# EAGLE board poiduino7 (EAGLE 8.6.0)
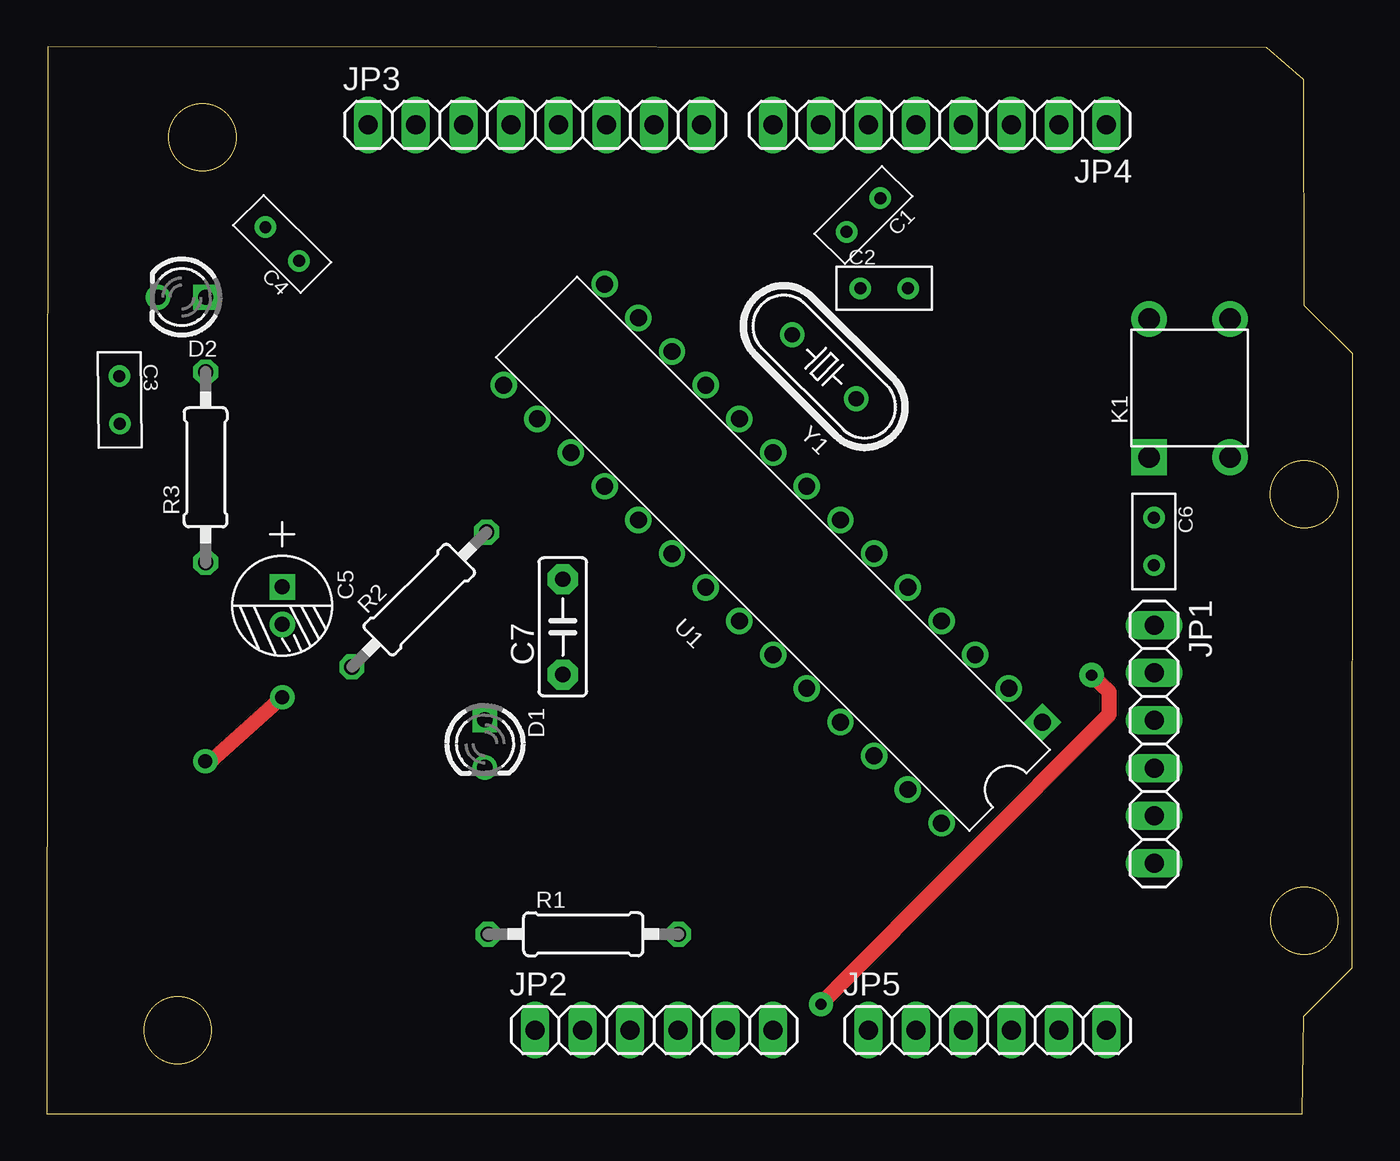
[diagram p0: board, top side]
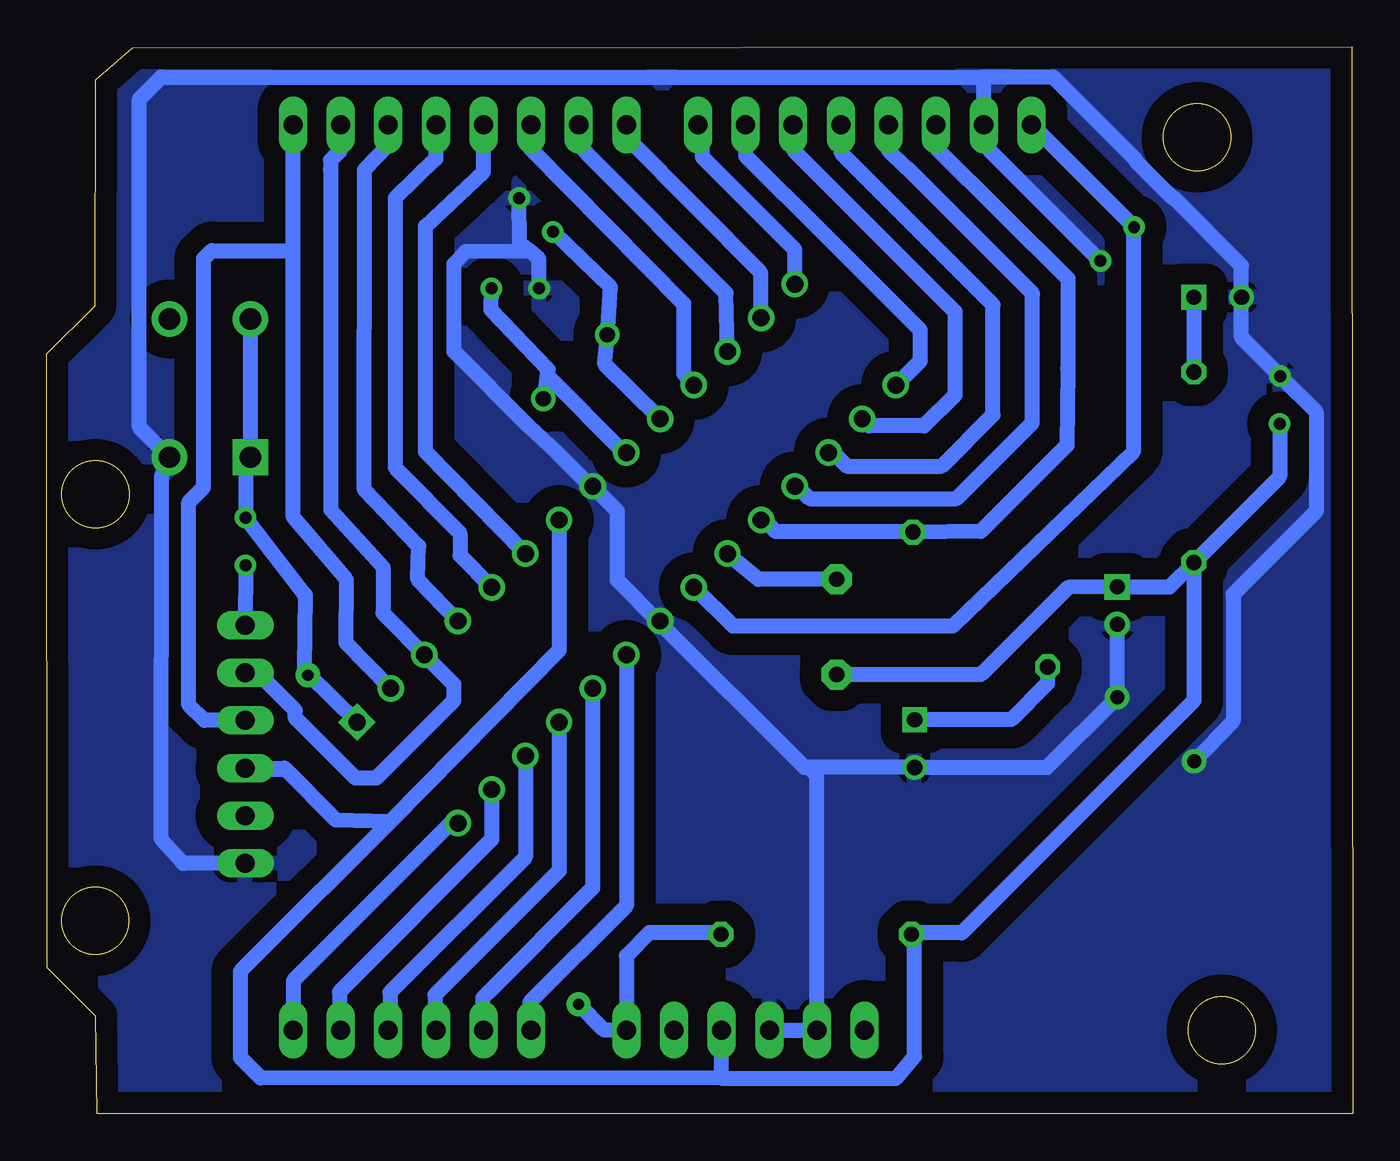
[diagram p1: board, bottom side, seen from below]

Size 69.63 x 56.88 mm. Coordinates in mm from the lower left corner, seen from the top.
Outline: 0,0.01 59.03,0.01 66.95,0 67.02,5.21 69.61,7.8 69.63,40.51 67.06,43.08 67.02,55.14 65.05,56.84 0.05,56.88 0,0.01
Outline: circle at 8.29,52.06 radius 1.8
Outline: circle at 6.98,4.47 radius 1.8
Outline: circle at 67.04,33.04 radius 1.8
Outline: circle at 67.05,10.3 radius 1.8
Copper layers (1*16): Top 0.035mm / dielectric 1.5mm / Bottom 0.035mm
Design rules "default": minimum track width 6mil, minimum drill 0.35mm, track to track 6mil, track to pad 6mil, pad to pad 6mil, via to via 6mil, smd to smd 6mil, copper to edge 40mil, drill to drill 6mil, minimum pad ring 10mil, minimum via ring 8mil, stop-mask expansion 4mil, vias tented up to drill 0mil, thermal gap 10mil

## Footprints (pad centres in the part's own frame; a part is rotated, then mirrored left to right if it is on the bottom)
CERAMIC-2.54 = drill 0.635 pad 1.143: 1 -1.27,0; 2 1.27,0
PC-D5.3MM = drill 0.8 pad 1.35 square: + -1,0 | drill 0.8 pad 1.35: - 1,0
C5B2.5 = drill 0.813 pad 1.6 octagon: 1 -2.54,0; 2 2.54,0
LED2-2.54-D3.0MM = drill 0.813 square: A -1.27,0 | drill 0.813: K 1.27,0
1X06 = drill 1.016 long: 1 -6.35,0; 2 -3.81,0; 3 -1.27,0; 4 1.27,0; 5 3.81,0; 6 6.35,0
1X08 = drill 1.016 long: 1 -8.89,0; 2 -6.35,0; 3 -3.81,0; 4 -1.27,0; 5 1.27,0; 6 3.81,0; 7 6.35,0; 8 8.89,0
SW4-6.0X6.0X5.0MM = drill 1.143 pad 1.905 square: 1 -3.683,2.159 | drill 1.143 pad 1.905: 2 -3.683,-2.159; 3 3.683,-2.159; 4 3.683,2.159
PR-D2.3XL6.5MM = drill 0.813 octagon: 1 -4.953,0; 2 5.207,0
DIP28-2.54-34.7X7.62MM = drill 0.9 pad 1.4 square: 1 -16.51,-3.81 | drill 0.9 pad 1.4: 2 -13.97,-3.81; 3 -11.43,-3.81; 4 -8.89,-3.81; 5 -6.35,-3.81; 6 -3.81,-3.81; 7 -1.27,-3.81; 8 1.27,-3.81; 9 3.81,-3.81; 10 6.35,-3.81; 11 8.89,-3.81; 12 11.43,-3.81; 13 13.97,-3.81; 14 16.51,-3.81; 15 16.51,3.81; 16 13.97,3.81; 17 11.43,3.81; 18 8.89,3.81; 19 6.35,3.81; 20 3.81,3.81; 21 1.27,3.81; 22 -1.27,3.81; 23 -3.81,3.81; 24 -6.35,3.81; 25 -8.89,3.81; 26 -11.43,3.81; 27 -13.97,3.81; 28 -16.51,3.81
HC49US = drill 0.813: 1 -2.413,0; 2 2.413,0

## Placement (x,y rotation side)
C1  18pf  [CERAMIC-2.54]  43.54,47.92 225 top
C2  18pf  [CERAMIC-2.54]  44.65,44.01 0 top
C3  0.1uf  [CERAMIC-2.54]  3.88,38.06 270.6 top
C4  0.1uf  [CERAMIC-2.54]  12.55,46.38 135 top
C5  1uf  [PC-D5.3MM]  12.55,27.09 270 top
C6  0.1uf  [CERAMIC-2.54]  59.04,30.52 270 top
C7  0.1uf  [C5B2.5]  27.51,25.96 90 top
D1  CX-G302DC  [LED2-2.54-D3.0MM]  23.36,19.74 270 top
D2  CX-G302DC  [LED2-2.54-D3.0MM]  7.2,43.54 180 top
JP1  [1X06]  59.05,19.71 270 top
JP2  [1X06]  32.38,4.47 0 top
JP3  [1X08]  26.03,52.73 0 top
JP4  [1X08]  47.62,52.73 180 top
JP5  [1X06]  50.16,4.47 0 top
K1  TS-1109  [SW4-6.0X6.0X5.0MM]  60.94,38.69 90 top
R1  10K  [PR-D2.3XL6.5MM]  28.48,9.58 0 top
R2  1K  [PR-D2.3XL6.5MM]  19.77,27.33 45 top
R3  1K  [PR-D2.3XL6.5MM]  8.47,34.34 90 top
U1  [DIP28-2.54-34.7X7.62MM]  38.73,29.87 135 top
Y1  16MHZ  [HC49US]  41.45,39.84 135 top

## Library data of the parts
C1-C4 C6 = Seeed-Capacitor
C5 = Seeed-Capacitor; MPN: KS 100uF/16V
C7 = capacitor-wima
D1 D2 = Seeed-LED; MPN: CX-G302DC
JP1-JP5 = pinhead
K1 = Seeed-OPL-Button; MPN: TS-1109
R1 = Seeed-Resistor; MPN: FHCFR-1/4W-103J
R2 R3 = Seeed-Resistor; MPN: FHCFR-1/4W-102J
U1 = Seeed-IC; MPN: ATMEGA328P-PU
Y1 = Seeed-Crystal Oscillator; MPN: HC-49US 16.000MHz

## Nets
A0: JP5.1 U1.23
A1: JP5.2 U1.24
A2: JP5.3 U1.25
A3: JP5.4 U1.26
A4-SDA: JP5.5 U1.27
A5-SCL: JP5.6 U1.28
AREF: C4.2 JP3.1 U1.21
AVCC: C7.2 U1.20
CTS: JP1.5
DTR: C6.2 JP1.1
GND: C1.1 C2.1 C3.1 C4.1 C5.- D1.K D2.K JP1.6 JP2.2 JP2.3 JP3.2 K1.2 U1.8 U1.22
N$3: D2.A R3.2
N$6: D1.A R2.1
N$34: JP2.1
N$38: JP2.5
PIN2: JP4.3 U1.4
PIN3: JP4.4 U1.5
PIN4: JP4.5 U1.6
PIN5: JP4.6 U1.11
PIN6: JP4.7 U1.12
PIN7: JP4.8 U1.13
PIN8: JP3.8 U1.14
PIN9: JP3.7 U1.15
PIN10: JP3.6 U1.16
PIN11: JP3.5 U1.17
PIN12: JP3.4 U1.18
PIN13: JP3.3 R2.2 U1.19
RESET: C6.1 JP2.6 K1.1 K1.4 R1.2 U1.1
RXD: JP1.3 JP4.1 U1.2
TXD: JP1.2 JP4.2 U1.3
VCC: C3.2 C5.+ C7.1 JP1.4 JP2.4 R1.1 R3.1 U1.7
XTAL1: C2.2 U1.9 Y1.1
XTAL2: C1.2 U1.10 Y1.2

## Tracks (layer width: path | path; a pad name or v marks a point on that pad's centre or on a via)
A0
  Bottom 0.813: U1.23 38.73,11.11 43.89,5.95 43.89,4.55 JP5.1
A1
  Bottom 0.813: U1.24 40.52,12.05 46.13,6.44 46.39,6.18 46.39,4.51 JP5.2
A2
  Bottom 0.813: U1.25 42.32,12.96 48.93,6.34 48.93,4.52 JP5.3
A3
  Bottom 0.813: U1.26 44.11,13.69 51.33,6.48 51.33,4.56 JP5.4
A4-SDA
  Bottom 0.813: U1.27 45.91,14.63 54.03,6.51 54.03,4.53 JP5.5
A5-SCL
  Bottom 0.813: U1.28 48.09,15.5 56.49,7.09 56.49,4.48 JP5.6
AREF
  Bottom 0.813: U1.21 33.05,26.02 21.33,26.02 11.68,35.33 11.68,47.25 C4.2 17.11,52.73 JP3.1
AVCC
  Bottom 0.813: C7.2 28.07,28.51 31.69,28.5 U1.20
DTR
  Bottom 0.813: C6.2 JP1.1
GND  (via drill 0.75 pad 1.3)
  Top 0.813: v12.55,22.21 8.68,18.74 8.6,18.75 v8.44,18.8
  Bottom 0.813: 19.67,55.27 19.68,54 JP3.2 19.37,52.42 19.37,51.38 13.47,45.48 C4.1 | JP2.3 JP2.2 28.58,4.48 28.58,18.05 28.99,18.47 | JP1.6 62.37,13.36 63.53,14.64 63.51,33.99 K1.2 64.71,36.62 64.71,54.1 63.54,55.27 19.67,55.27 | 37.04,26.27 U1.22 36.93,26.11 | 37.04,26.27 39.2,28.44 39.2,32.14 U1.8 40.63,33.46 42.39,35.22 43.95,36.66 47.92,40.65 47.93,45.3 47.31,45.98 43.88,46.02 43.4,45.58 | C2.1 43.4,45.58 | 43.4,45.58 44.41,46.42 C1.1 | C5.- v12.55,22.21 16.29,18.47 D1.K 28.99,18.47 | 19.67,55.27 15.97,55.27 11.51,50.81 11.51,50.73 9.62,48.84 9.54,48.84 5.93,45.23 D2.K 5.93,41.4 C3.1 1.95,37.42 1.95,32.12 6.37,27.71 6.37,20.97 v8.44,18.8 | 28.99,18.47 29.23,18.47 37.04,26.27
  pour Bottom (isolate 1.143): -0.78,58.59 70.78,58.59 70.78,-2.57 -0.94,-2.57 -0.94,58.59
N$3
  Bottom 0.813: D2.A R3.2
N$6
  Bottom 0.813: R2.1 16.27,22.96 18.2,21.02 23.34,21.02 D1.A
PIN2
  Bottom 0.813: U1.4 49.86,28.51 49.81,30.27 52.71,33.29 52.69,50.33 51.43,51.63 JP4.3
PIN3
  Bottom 0.813: JP4.4 48.89,52.76 48.89,50.91 51.05,48.82 51.06,34.45 47.61,30.96 47.61,29.78 U1.5
PIN4
  Bottom 0.813: U1.6 49.44,35.31 49.44,47.33 46.35,50.22 JP4.5
PIN5
  Bottom 0.813: JP4.6 43.82,51.41 35.68,43.19 35.67,39.48 U1.11
PIN6
  Bottom 0.813: U1.12 33.4,43.76 40.76,51.12 41.02,51.42 41.36,52.26 41.18,52.64 JP4.7
PIN7
  Bottom 0.813: U1.13 31.56,44.83 38.58,51.92 38.61,52.61 JP4.8
PIN8
  Bottom 0.813: U1.14 29.75,46.08 34.68,51.01 34.68,52.49 JP3.8
PIN9
  Bottom 0.813: JP3.7 32.38,51.07 30.33,49.02 30.3,49.02 23.07,41.8 23.07,40.13 U1.15
PIN10
  Bottom 0.813: JP3.6 29.84,51.4 21.21,42.77 21.21,38.32 22.85,36.67 25.78,36.67 U1.16
PIN11
  Bottom 0.813: U1.17 27.69,35.26 26.97,34.53 21.9,34.53 19.17,37.27 19.17,43.13 27.28,51.24 27.28,52.71 JP3.5
PIN12
  Bottom 0.813: JP3.4 24.76,51.38 23.83,50.45 23.8,50.45 17.09,43.75 | 17.09,43.75 17.05,43.71 | U1.18 29.62,33.46 28.96,32.8 21.13,32.8 17.09,36.83 17.09,43.75
PIN13
  Bottom 0.813: U1.19 31.39,31.66 30.78,31.05 23.43,31.06 R2.2 19.83,31.05 15.24,35.64 15.19,39.72 15.18,44.52 22.22,51.51 JP3.3
RESET  (via drill 0.6 pad 1.3)
  Top 0.813: v41.28,5.85 41.47,6.05 56.66,21.3 56.66,22.48 v55.71,23.39
  Bottom 0.813: U1.1 55.7,23.43 | 55.7,23.43 55.89,23.74 55.84,27.65 55.9,27.74 C6.1 59.04,34.75 K1.1 K1.4 | R1.2 34.06,9.66 37.51,9.66 38.73,8.44 JP2.6 39.92,4.47 v41.28,5.85 | v55.71,23.39 v55.7,23.37 55.7,23.43
RXD
  Bottom 0.813: U1.2 53.68,25.12 53.66,28.47 56.49,31.81 56.51,41.15 56.51,46.15 | 56.51,46.15 JP4.1 | JP1.3 61.24,20.98 62.06,21.8 62.06,32.62 61.27,33.4 61.27,45.59 60.84,46.02 56.63,46.02 56.51,46.15
TXD
  Bottom 0.813: JP4.2 53.95,51.4 54.51,50.84 54.51,50.34 54.5,32.2 51.71,29.15 51.71,26.7 51.43,26.43 U1.3 47.93,22.91 47.93,22.03 52.07,17.9 53.17,17.9 56.39,21.11 56.39,21.51 58.39,23.52 JP1.2
VCC
  Bottom 0.813: JP2.4 33.67,1.91 | 33.67,1.91 24.36,1.89 23.36,3.07 23.36,9.3 R1.1 23.45,9.66 20.84,9.66 8.47,22.03 R3.1 | U1.7 42.32,24.72 51.33,15.57 | 51.33,15.57 54.21,15.66 56.86,18.34 | 56.86,18.34 59.42,18.34 59.56,18.19 | JP1.4 56.96,18.44 56.86,18.34 | 51.33,15.57 50.62,16.3 59.32,7.6 59.32,3.01 58.23,1.93 33.67,1.91 | C7.1 25.2,23.42 19.83,23.41 15.16,28.07 C5.+ 9.76,28.09 R3.1 | C3.2 3.89,33.97 R3.1
XTAL1
  Bottom 0.813: U1.9 38.86,35.26 42.94,39.35 43.13,38.25 Y1.1 43.07,38.29 42.9,39.69 45.95,42.88 C2.2
XTAL2
  Bottom 0.813: U1.10 39.88,39.97 Y1.2 39.58,44.07 C1.2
